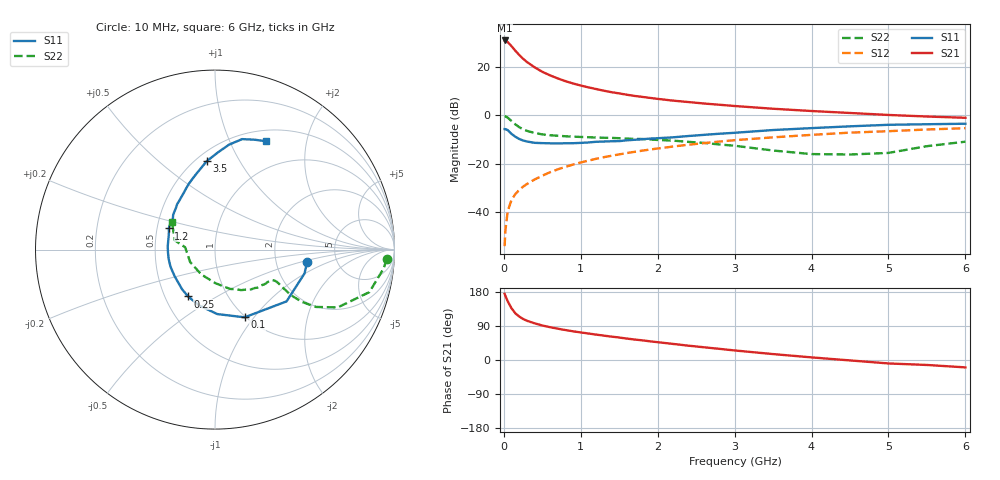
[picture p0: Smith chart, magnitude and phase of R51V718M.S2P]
! SIEMENS Small Signal Semiconductors
! BFR183
! Si NPN RF Bipolar Junction Transistor in SOT23
! VCE = 1.75 V  IC = 18 mA
! Common Emitter S-Parameters:  May  1996
# GHz  S  MA  R  50
!  f  S11  S21  S12  S22
! GHz  MAG  ANG  MAG  ANG  MAG  ANG  MAG  ANG
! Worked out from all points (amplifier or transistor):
!   36 points, 10 MHz to 6 GHz, reference 50 ohm
!   highest |S21| = 30.8 dB at 10 MHz (marker M1)
!   |S21| within 3 dB of that: start of sweep to 117 MHz
!   unconditionally stable (mu >= 1): 524.2 MHz to 2.414 GHz
!   at 250 MHz: K = 0.80, MSG = 26.4 dB, |S12| = -29.5 dB
!   at 1.4 GHz: K = 1.05, MAG = 11.7 dB, |S12| = -16.7 dB
!   at 6 GHz: K = 0.91, MSG = 2.1 dB, |S12| = -5.4 dB
!   S11 on the Smith chart (normalised r, x): 10 MHz: 3.02, -0.59; 100 MHz: 0.99, -0.90; 250 MHz: 0.65, -0.38; 1.2 GHz: 0.58, +0.15; 3.5 GHz: 0.56, +0.74; 6 GHz: 0.63, +1.37
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0.01  0.5178 -7.9  34.67 174.7  0.002 90.5  0.959 -3.1
0.02  0.5163 -14.9  34.2 169.4  0.0042 84.0  0.9447 -6.5
0.05  0.4922 -35.9  32.16 155.0  0.0105 75.5  0.8921 -15.4
0.1  0.4117 -66.4  26.44 136.4  0.018 68.5  0.7562 -25.2
0.15  0.3594 -88.0  21.25 123.2  0.0238 66.2  0.6469 -29.6
0.2  0.3235 -105.8  17.44 114.6  0.0288 65.8  0.5666 -31.0
0.25  0.3011 -119.9  14.56 108.3  0.0336 66.6  0.5115 -31.0
0.3  0.287 -129.8  12.49 103.6  0.0382 67.6  0.4765 -30.5
0.4  0.2694 -146.6  9.695 96.8  0.0473 68.8  0.4297 -29.2
0.5  0.2657 -158.9  7.84 91.1  0.0566 69.9  0.4022 -28.0
0.6  0.2634 -168.3  6.625 86.6  0.0668 70.1  0.3866 -27.5
0.7  0.2624 -176.2  5.736 82.7  0.0764 70.1  0.377 -27.5
0.8  0.2639 176.4  5.032 79.1  0.086 69.5  0.3679 -27.8
0.9  0.2647 170.6  4.504 75.7  0.0961 69.5  0.361 -28.1
1.1  0.274 159.7  3.741 69.9  0.1158 68.5  0.3516 -30.2
1.2  0.2832 155.4  3.457 67.0  0.1265 67.8  0.3463 -31.2
1.6  0.3037 140.1  2.639 56.5  0.166 64.0  0.329 -36.8
2.2  0.3499 121.9  1.996 42.4  0.2261 57.7  0.299 -47.9
3.5  0.4944 95.4  1.358 15.6  0.3496 40.9  0.1871 -89.3
4.5  0.5897 82.4  1.111 -1.1  0.437 27.9  0.1549 -153.5
5.5  0.651 70.1  0.939 -13.1  0.5074 16.0  0.2299 167.1
6  0.6669 64.9  0.884 -19.5  0.5396 8.3  0.2846 147.4
